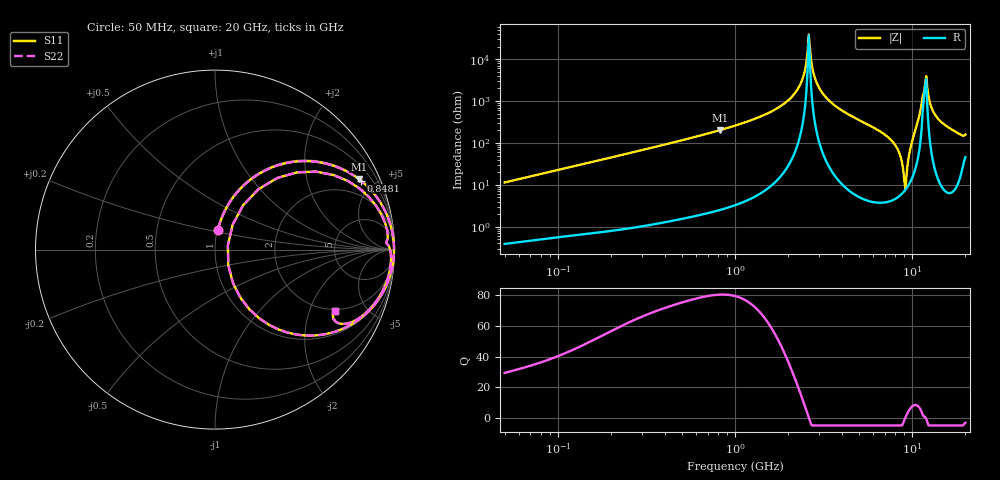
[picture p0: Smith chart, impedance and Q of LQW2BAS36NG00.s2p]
!Murata Part Number: LQW2BAS36NG00
!These Parameters are Measured in Series Mode Connection
!  o--[Z]--o
!Port1  Port2
!  o-------o
!Freq. Start=50[MHz] Stop=20[GHz], 401[Steps]
# Hz S RI R 50
!Freq.(Hz) S11(Real) S11(Imag) S21(Real) S21(Imag) S12(Real) S12(Imag) S22(Real) S22(Imag)
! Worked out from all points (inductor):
!   401 points, 50 MHz to 20 GHz, reference 50 ohm
!   read as one part in series: L = 36.1 nH near 51.52 MHz
!   highest Q = 80.5 at 823.1 MHz (marker M1), where L = 39.1 nH
!   self-resonance near 2.608 GHz
!   S11 on the Smith chart (normalised r, x): 50 MHz: 1.01, +0.23; 848.1 MHz: 1.05, +4.19; 20 GHz: 1.92, -3.02
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5e7  0.0165 0.1115  0.9835 -0.1115  0.9835 -0.1115  0.0165 0.1115
1.364002e8  0.0913 0.2776  0.9087 -0.2776  0.9087 -0.2776  0.0913 0.2776
3.721004e8  0.4189 0.4863  0.5811 -0.4863  0.5811 -0.4863  0.4189 0.4863
8.230629e8  0.8006 0.3934  0.1994 -0.3934  0.1994 -0.3934  0.8006 0.3934
8.480927e8  0.8118 0.3847  0.1882 -0.3847  0.1882 -0.3847  0.8118 0.3847
1e9  0.8669 0.3335  0.1331 -0.3335  0.1331 -0.3335  0.8669 0.3335
1.932977e9  0.9859 0.1061  0.0141 -0.1061  0.0141 -0.1061  0.9859 0.1061
2.348516e9  0.9961 0.038  0.0039 -0.038  0.0039 -0.038  0.9961 0.038
2.608132e9  0.9976 0.000867  0.00242 -0.000867  0.00242 -0.000867  0.9976 0.000867
2.728004e9  0.9974 -0.0152  0.00265 0.0152  0.00265 0.0152  0.9974 -0.0152
2.940159e9  0.9958 -0.0423  0.00423 0.0423  0.00423 0.0423  0.9958 -0.0423
3.466789e9  0.9865 -0.1039  0.0135 0.1039  0.0135 0.1039  0.9865 -0.1039
5.683258e9  0.8744 -0.3238  0.1256 0.3238  0.1256 0.3238  0.8744 -0.3238
7.442007e9  0.6203 -0.47  0.3797 0.47  0.3797 0.47  0.6203 -0.47
8.389408e9  0.3018 -0.4197  0.6982 0.4197  0.6982 0.4197  0.3018 -0.4197
9.041845e9  0.0745 -0.0888  0.9255 0.0888  0.9255 0.0888  0.0745 -0.0888
9.316812e9  0.0981 0.138  0.9019 -0.138  0.9019 -0.138  0.0981 0.138
9.745021e9  0.3463 0.3987  0.6537 -0.3987  0.6537 -0.3987  0.3463 0.3987
1.066139e10  0.8579 0.2928  0.1421 -0.2928  0.1421 -0.2928  0.8579 0.2928
1.183995e10  0.9689 0.02  0.0311 -0.02  0.0311 -0.02  0.9689 0.02
1.417136e10  0.9208 -0.2537  0.0792 0.2537  0.0792 0.2537  0.9208 -0.2537
2e10  0.6695 -0.3425  0.3305 0.3425  0.3305 0.3425  0.6695 -0.3425
